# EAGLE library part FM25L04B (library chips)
IC FRAM 4KBIT 10MHZ
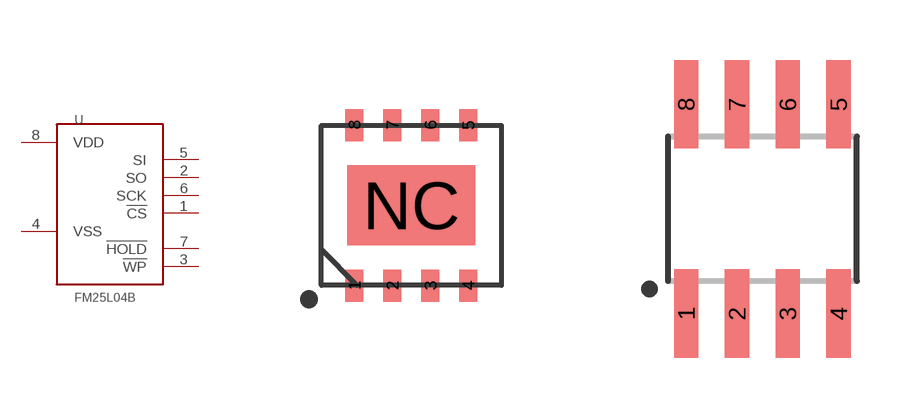
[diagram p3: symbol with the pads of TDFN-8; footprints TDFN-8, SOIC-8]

Designator prefix U

## FM25L04B-DG (DIGIKEY: FM25L04B-DGRA-ND)  [TDFN-8]
1  !CS
2  SO
3  !WP
4  VSS
5  SI
6  SCK
7  !HOLD
8  VDD

## FM25L04B-G  [SOIC-8]
Pads as for TDFN-8

## Footprint TDFN-8 (pad centres in mm)
smd 0.45 x 0.8: 1 -1.425,-2.007; 2 -0.475,-2.007; 3 0.475,-2.007; 4 1.425,-2.007; 5 1.425,2.007; 6 0.475,2.007; 7 -0.475,2.007; 8 -1.425,2.007
smd 3.2 x 2: NC 0,0

## Footprint SOIC-8 (pad centres in mm)
smd 0.61 x 2.21: 1 -1.905,-2.616; 2 -0.635,-2.616; 3 0.635,-2.616; 4 1.905,-2.616; 5 1.905,2.616; 6 0.635,2.616; 7 -0.635,2.616; 8 -1.905,2.616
